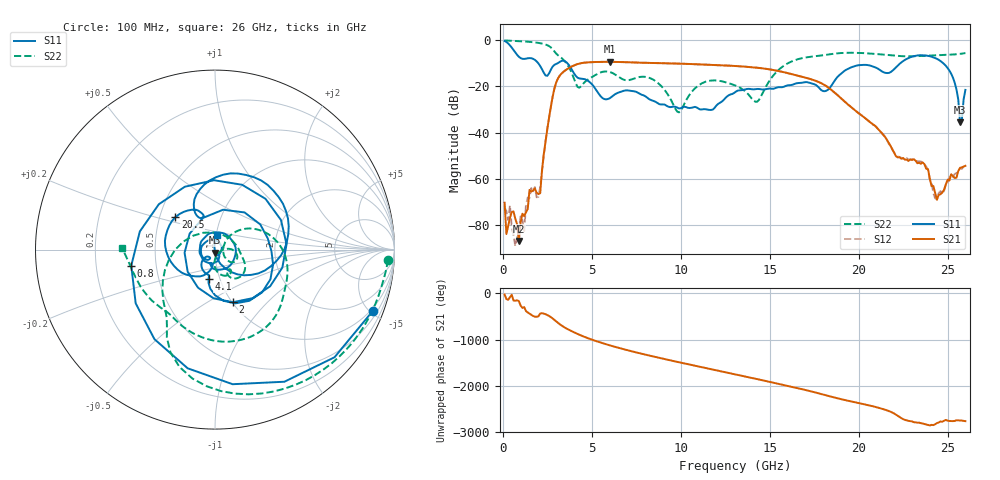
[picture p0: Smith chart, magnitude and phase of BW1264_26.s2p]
!Keysight Technologies,N5245B,MY57181159,A.13.60.06
!Date: Friday, December 18, 2020 23:53:18
!Correction: S11(Full 2 Port(1,2))
!S21(Full 2 Port(1,2))
!S12(Full 2 Port(1,2))
!S22(Full 2 Port(1,2))
!S2P File: Measurements: S11, S21, S12, S22:
# Hz S  dB  R 50
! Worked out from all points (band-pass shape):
!   260 points, 100 MHz to 26 GHz, reference 50 ohm
!   highest |S21| = -9.49 dB at 6 GHz (marker M1); lowest = -86.7 dB at 900 MHz (marker M2)
!   |S21| within 3 dB of the highest: 3.648 GHz to 14.76 GHz (11.11 GHz wide, 121 % of centre)
!   lowest |S11| = -35.6 dB at 25.7 GHz (marker M3), VSWR 1.03, Z = 50 - j1.65 ohm
!   |S11| at or under -10 dB: 1.979 GHz to 3.109 GHz (1.13 GHz wide, 44.4 % of centre); 3.614 GHz to 22.36 GHz (18.75 GHz wide, 144 % of centre); 24.73 GHz to end of sweep
!   |S22| runs from -31.3 to -0.3 dB; largest |S21 - S12| = 0.00054
!   S11 on the Smith chart (normalised r, x): 100 MHz: 0.84, -5.17; 800 MHz: 0.36, -0.08; 2 GHz: 1.01, -0.65; 4.1 GHz: 0.88, -0.30; 20.5 GHz: 0.60, +0.24; 26 GHz: 1.01, +0.17
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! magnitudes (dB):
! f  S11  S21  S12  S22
! 100 MHz  -0.5  -70.2  -72.3  -0.3
! 200 MHz  -1.0  -83.7  -73.8  -0.4
! 800 MHz  -6.5  -79.5  -85.4  -0.6
! 900 MHz  -7.3  -86.7  -82.5  -0.6
! 1.6 GHz  -8.0  -65.4  -63.9  -1.0
! 2 GHz  -10.2  -66.5  -67.6  -1.4
! 2.9 GHz  -10.8  -21.0  -21.0  -5.1
! 4.1 GHz  -15.6  -10.8  -10.7  -18.8
! 4.5 GHz  -16.8  -10.0  -10.0  -19.1
! 6 GHz  -25.3  -9.5  -9.5  -13.9
! 8.8 GHz  -27.8  -10.1  -10.1  -19.2
! 9.9 GHz  -29.6  -10.3  -10.3  -31.3
! 11.2 GHz  -30.0  -10.6  -10.6  -18.7
! 13.1 GHz  -22.3  -11.3  -11.3  -19.8
! 14.3 GHz  -21.2  -12.1  -12.1  -26.7
! 17.4 GHz  -18.9  -17.2  -17.2  -7.2
! 20.5 GHz  -10.9  -34.6  -34.6  -5.9
! 21.7 GHz  -14.3  -44.6  -44.9  -6.6
! 24.6 GHz  -9.2  -66.6  -65.2  -6.6
! 25.4 GHz  -18.5  -59.5  -57.8  -6.3
! 25.7 GHz  -35.6  -55.2  -55.2  -6.1
! 26 GHz  -21.6  -54.3  -54.3  -5.7
